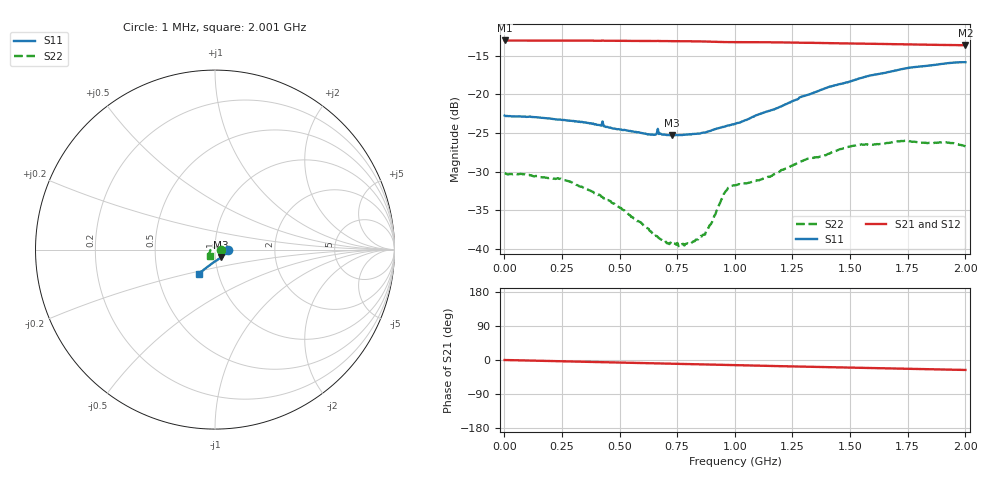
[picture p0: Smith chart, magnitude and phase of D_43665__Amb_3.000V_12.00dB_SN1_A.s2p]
! device id: 43665_
! dir: \\malibu\benchdata\1_engineers\tn_data\43665_75ohm\new\sparar\43665_\amb\3p000v\12p00db
! Serial: 1
! Insertion: A
! Temp: Amb
! VDD: 3.000V
! Attenuation Step: 12.00dB
! IDD: 1.450042e+00mA
! FILE NAME
! DATE 03-27-2009 08:36:19
! CORRECTED  DATA
#  Hz  S  RI  R  75
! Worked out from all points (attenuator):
!   401 points, 1 MHz to 2.001 GHz, reference 75 ohm
!   highest |S21| = -13.03 dB at 1 MHz (marker M1); lowest = -13.7 dB at 2.001 GHz (marker M2)
!   lowest |S11| = -25.3 dB at 726 MHz (marker M3), VSWR 1.11, Z = 79.8 - j6.95 ohm
!   |S11| at or under -10 dB: start of sweep to end of sweep
!   |S22| runs from -39.6 to -26.0 dB; largest |S21 - S12| = 0.00061
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1000000  0.0729 -0.000774  0.223 -0.000342  0.223 -0.000365  0.0308 -0.000154
2.41e8  0.0674 -0.0137  0.2222 -0.0122  0.2223 -0.0124  0.0265 0.0101
3.36e8  0.0637 -0.0193  0.2217 -0.0171  0.2218 -0.0173  0.0216 0.0133
4.16e8  0.0585 -0.0235  0.2211 -0.0212  0.2212 -0.0214  0.0174 0.014
5.11e8  0.0515 -0.0287  0.2202 -0.0265  0.2203 -0.0264  0.0114 0.014
6.31e8  0.041 -0.0369  0.2187 -0.0326  0.2187 -0.0326  0.00251 0.0129
6.71e8  0.0385 -0.0398  0.2184 -0.0347  0.2183 -0.0346  0.000625 0.0117
7.01e8  0.0352 -0.042  0.2179 -0.0363  0.2179 -0.0362  -0.00113 0.0111
7.26e8  0.0327 -0.0434  0.2175 -0.0376  0.2176 -0.0375  -0.0025 0.0104
7.91e8  0.0262 -0.0483  0.2165 -0.0412  0.2165 -0.0411  -0.00761 0.00772
8.66e8  0.0176 -0.0537  0.2149 -0.0455  0.2149 -0.0452  -0.0123 0.0016
8.96e8  0.0142 -0.0565  0.2139 -0.047  0.214 -0.0468  -0.0144 -0.000917
9.61e8  0.00683 -0.0618  0.2119 -0.0494  0.2121 -0.0491  -0.0236 -0.00262
9.81e8  0.00484 -0.0632  0.2117 -0.05  0.2119 -0.0497  -0.0252 -0.00194
1.001e9  0.00223 -0.0645  0.2116 -0.0508  0.2118 -0.0506  -0.0257 -0.00198
1.151e9  -0.0154 -0.0768  0.2089 -0.0583  0.2092 -0.0581  -0.0276 -0.0099
1.336e9  -0.0392 -0.0939  0.2045 -0.067  0.2049 -0.0668  -0.0321 -0.0221
1.511e9  -0.058 -0.1078  0.1995 -0.0745  0.2 -0.0746  -0.0341 -0.0316
1.671e9  -0.0725 -0.1195  0.1952 -0.0808  0.1954 -0.081  -0.033 -0.0357
1.741e9  -0.0778 -0.1248  0.1932 -0.0834  0.1935 -0.0836  -0.0321 -0.0385
1.916e9  -0.0882 -0.1318  0.1885 -0.0891  0.1886 -0.0891  -0.0304 -0.0385
2.001e9  -0.0907 -0.1335  0.1863 -0.0917  0.1859 -0.0921  -0.0277 -0.0369
